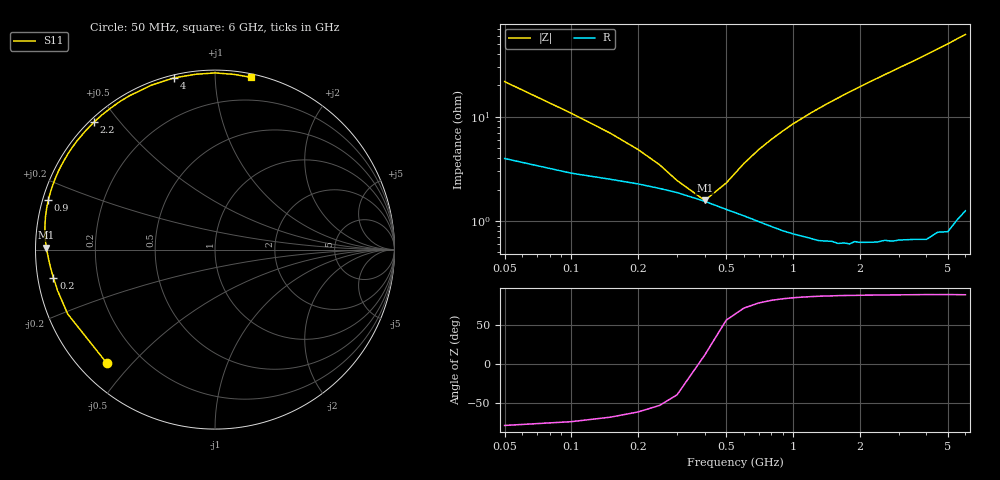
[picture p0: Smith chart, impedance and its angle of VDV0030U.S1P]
! Infineon Technologies  Discrete & RF Semiconductors
! BBY 55-03
! Si Tuning Diode in SOD323
! VR =
! S-Parameters:  June  1999
# GHz  S  MA  R  50
!  f  S11
! GHz  MAG  ANG
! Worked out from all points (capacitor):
!   34 points, 50 MHz to 6 GHz, reference 50 ohm
!   read as one part to ground: C = 142 pF near 50 MHz
!   lowest |Z| = 1.57 ohm at 400 MHz (marker M1)
!   series resonance near 383.7 MHz, so ESL is about 1.2 nH
!   S11 on the Smith chart (normalised r, x): 50 MHz: 0.08, -0.43; 200 MHz: 0.05, -0.09; 900 MHz: 0.02, +0.14; 2.2 GHz: 0.01, +0.43; 4 GHz: 0.01, +0.79; 6 GHz: 0.02, +1.23
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0.05  0.8742 -133.5
0.1  0.8957 -156.4
0.15  0.9059 -165.2
0.2  0.9139 -170.2
0.25  0.9215 -173.6
0.3  0.928 -176.4
0.4  0.9402 179.3
0.5  0.9498 175.6
0.6  0.9564 172.3
0.7  0.9617 169.2
0.8  0.9658 166.3
0.9  0.969 163.5
1  0.9712 160.7
1.2  0.9743 155.6
1.4  0.9763 150.8
1.6  0.978 146.3
1.8  0.9788 141.8
2.2  0.9792 133.6
2.4  0.9796 129.9
2.6  0.9795 126.1
2.8  0.9805 122.6
3  0.9807 119.1
3.5  0.9821 111.1
4  0.9838 103.5
4.5  0.9829 96.3
5  0.9844 89.9
5.5  0.982 83.6
6  0.9804 78.1
